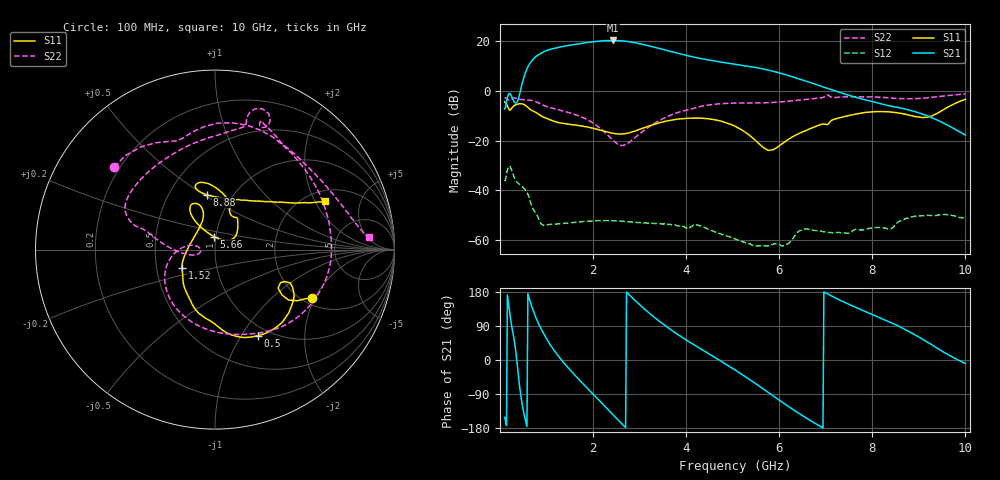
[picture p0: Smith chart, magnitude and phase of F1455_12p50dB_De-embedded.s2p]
! Integrated Device Technology
! Corporate Headquarters
! 6024 Silver Creek Valley Road
! San Jose, CA 95138  USA
! Phone:  1-408-284-8200
! Toll Free:  1-800-223-1366
! Webpage:  http://www.idt.com/
! Timing and RF Division
! 515 Groton Road, Suite 102
! Westford, MA 01886-6024
! Device:  F1455
! Description: 6-bit 0.5 dB Transmit Variable Gain Amplifier
! Frequency:  1400.0 -  2300.00 MHz
! Package:  6x6 mm Thin QFN Plastic Package: 28 pin
! State:  25
! Atten State:  12.5 dB
! Voltage:  +5.00 Volts
! Current:  217.650 mA
! Data:  The device was measured on a the F1455 evaluation board which has
!  individual transmission lines to the RF pins.  Data was collected
!  using a calibrated network analyzer.  The evaluation board was
!  de-embedded using a TRL calibration technique.
!  The reference plane is the edge of the package pin.
!  Pin  1 = CSb
!  Pin  2 = DATA
!  Pin  3 = CLK
!  Pin  4 = RSET
!  Pin  5 = GND
!  Pin  6 = RFIN  = Port 1
!  Pin  7 = GND
!  Pin  8 = NC
!  Pin  9 = NC
!  Pin 10 = NC
!  Pin 11 = NC
!  Pin 12 = NC
!  Pin 13 = NC
!  Pin 14 = /STBY
!  Pin 15 = GND
!  Pin 16 = RFOUT  = Port 2
!  Pin 17 = GND
!  Pin 18 = NC
!  Pin 19 = NC
!  Pin 20 = NC
!  Pin 21 = GND
!  Pin 22 = NC
!  Pin 23 = GND
!  Pin 24 = NC
!  Pin 25 = NC
!  Pin 26 = NC
!  Pin 27 = GND
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# GHz S dB R 50
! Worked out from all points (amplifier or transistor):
!   496 points, 100 MHz to 10 GHz, reference 50 ohm
!   highest |S21| = 20.2 dB at 2.42 GHz (marker M1)
!   |S21| within 3 dB of that: 1.204 GHz to 3.38 GHz (2.176 GHz wide, 95 % of centre)
!   unconditionally stable (mu >= 1): start of sweep to end of sweep
!   at 1.74 GHz: K = 20.72, MAG = 19.6 dB, |S12| = -52.5 dB
!   at 5.06 GHz: K = 90.80, MAG = 12.5 dB, |S12| = -59.5 dB
!   at 10 GHz: K = 197.76, MAG = -9.3 dB, |S12| = -51.2 dB
!   S11 on the Smith chart (normalised r, x): 100 MHz: 2.24, -1.90; 500 MHz: 0.88, -1.19; 1.52 GHz: 0.68, -0.15; 5.66 GHz: 0.98, +0.14; 8.88 GHz: 0.76, +0.52; 10 GHz: 2.47, +2.44
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0.1  -4.38 -26.5  -7.31 -151.4  -36.21 45.6  -2.79 140.7
0.38  -5.34 -40.4  -4.16 -21.8  -36.97 -113.5  -3.17 57.1
0.5  -5.42 -63.5  4.52 -131.7  -38.88 -151.7  -3.60 27.8
0.68  -7.85 -92.1  11.93 142.3  -46.07 145.3  -3.86 -13.8
0.8  -9.02 -107.4  14.14 103.9  -50.05 127.9  -4.59 -41.4
0.94  -10.59 -121.1  15.64 69.5  -53.95 124.5  -5.88 -67.7
1.22  -12.61 -140.1  17.26 15.9  -53.52 97.5  -7.44 -107.1
1.52  -13.53 -150.9  18.35 -28.2  -52.99 68.6  -8.95 -138.4
1.76  -14.13 -158.1  19.07 -59.7  -52.49 50.5  -10.57 -158.2
2.1  -15.53 -171.6  19.88 -102.5  -52.12 28.7  -14.27 178.5
2.42  -17.06 165.4  20.19 -143.2  -52.14 10.4  -19.73 169.3
2.6  -17.34 147.6  20.06 -166.0  -52.37 1.4  -21.93 -179.1
2.8  -16.75 128.9  19.62 169.3  -52.60 -7.5  -20.37 -165.6
3.08  -14.96 112.7  18.58 137.2  -53.10 -18.2  -16.09 -170.1
3.4  -12.98 107.3  17.09 104.6  -53.33 -29.7  -12.23 178.3
4.1  -10.96 114.7  13.76 45.2  -54.51 -48.2  -7.37 163.9
5.06  -14.32 124.7  10.64 -26.9  -59.53 -91.4  -4.93 148.8
5.66  -22.79 93.5  8.73 -76.6  -62.38 -87.1  -4.84 124.5
6.7  -14.97 44.8  3.09 -162.1  -55.82 -135.7  -3.23 78.6
8.36  -8.46 106.3  -6.03 100.6  -55.46 156.6  -2.84 62.7
8.88  -10.18 98.6  -8.22 69.0  -50.54 141.7  -3.19 42.2
10  -3.46 23.8  -17.80 -9.1  -51.21 66.4  -1.29 4.7
